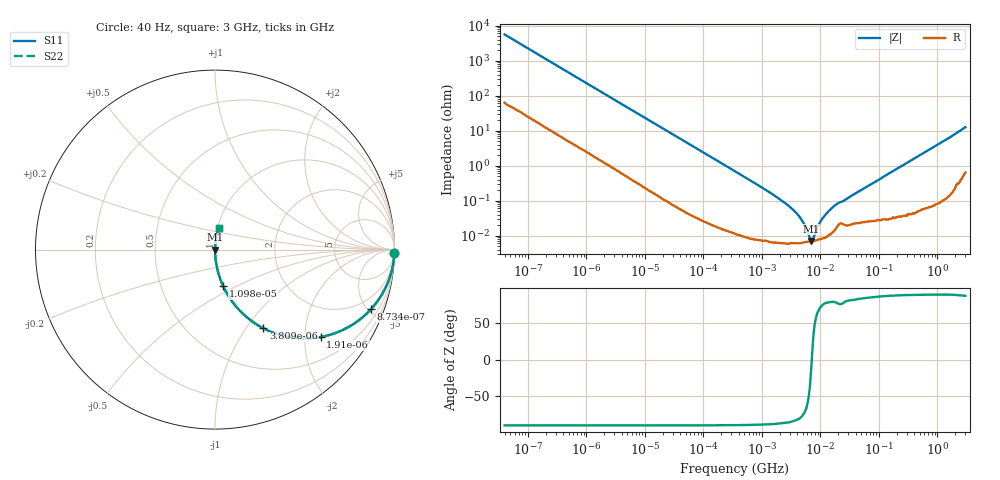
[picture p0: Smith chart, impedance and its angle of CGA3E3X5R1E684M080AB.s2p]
! S-parameter Generated by TDK Corporation
! Copyright(C) 2015 TDK Corporation.
! All Rights Reserved.
! TDK P/N: CGA3E3X5R1E684M080AB (Multilayer Ceramic Chip Capacitors)
! Property: C=680nF
! Size(LxWxT): 1.6x0.8x0.8mm, 0.063x0.031x0.031inches
! Model Type: s2p (Touchstone File Format Version 1.0)
! Frequency: DC=Yes Start=0.00004MHz Stop=3000MHz 396points Log-sweep
! Note: This model was converted from impedance.
! Model Generated on Jun. 23, 2015
! Hash(MD5):
! Port Assignments:
!  1 ---| |--- 2
! Applicable Conditions:
!  Temperature = 25 degC
!  DC Bias Voltage = 0 V
!  Small Signal Operation
! Terms and conditions regarding TDK Simulation Models
! (1)This simulation model is being provided solely for informational purposes. Please refer to the specifications of the products in terms of detailed characteristics of such products.
! (2)In no event shall TDK Corporation of any of its subsidiaries be liable for any loss or damage arising, directly or indirectly,
!  From any information contained in this simulation model, including, but not limited to loss or damages arising from any inaccuracies, omissions or errors in connection with such information.
! (3)Any and all copyrights on this simulation model are owned by TDK Corporation.
!  Duplication or redistribution of this simulation model without prior written permission from TDK Corporation is prohibited.
! (4)This simulation model is subject to any modification or change without any prior notice.
! (5)Neither TDK Corporation nor any of its subsidiaries shall make any warranty, express or implied,
!  Including but not limited to the correctness, implied warranties of merchantability and fitness for a particular purpose with respect to this simulation models.
! (6)The use of this simulation model shall be deemed to have consented to the terms and conditions hereof.
# MHz S MA R 50
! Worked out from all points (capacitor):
!   395 points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, 40 Hz to 3 GHz, reference 50 ohm
!   read as one part in series: C = 710 nF near 41.88 Hz
!   lowest |Z| = 6.98 mohm at 6.899 MHz (marker M1)
!   series resonance near 7.107 MHz, so ESL is about 710 pH
!   S11 on the Smith chart (normalised r, x): 40 Hz: open; 873.4 Hz: 1.06, -5.22; 1.91 kHz: 1.03, -2.40; 3.809 kHz: 1.01, -1.21; 10.98 kHz: 1.00, -0.42; 3 GHz: 1.01, +0.25
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4e-05  0.9996 -1.0  0.01783 88.3  0.01783 88.3  0.9996 -1.0
0.0002407527  0.9932 -6.1  0.1057 83.3  0.1057 83.3  0.9932 -6.1
0.000834128  0.9358 -20.0  0.3426 69.4  0.3426 69.4  0.9358 -20.0
0.000873414  0.9305 -20.9  0.3565 68.5  0.3565 68.5  0.9305 -20.9
0.001909884  0.7641 -39.6  0.6369 49.8  0.6369 49.8  0.7641 -39.6
0.003809071  0.515 -58.4  0.8519 31.0  0.8519 31.0  0.515 -58.4
0.006319477  0.3426 -69.4  0.936 20.0  0.936 20.0  0.3426 -69.4
0.01097819  0.2069 -77.5  0.9763 11.9  0.9763 11.9  0.2069 -77.5
0.01739424  0.133 -81.8  0.9898 7.6  0.9898 7.6  0.133 -81.8
0.3464102  0.006903 -88.7  0.9999 0.4  0.9999 0.4  0.006903 -88.7
2.877491  0.0007041 -85.2  0.9999 0.0  0.9999 0.0  0.0007041 -85.2
4.354128  0.0003502 -80.0  0.9999 0.0  0.9999 0.0  0.0003502 -80.0
5.480732  0.0001896 -69.9  0.9999 0.0  0.9999 0.0  0.0001896 -69.9
6.292177  0.0001072 -50.5  0.9999 0.0  0.9999 0.0  0.0001072 -50.5
6.898837  6.976e-05 -16.4  0.9999 0.0  0.9999 0.0  6.976e-05 -16.4
7.22376  6.992e-05 9.1  0.9999 -0.0  0.9999 -0.0  6.992e-05 9.1
7.920238  0.0001045 47.3  0.9999 -0.0  0.9999 -0.0  0.0001045 47.3
9.092863  0.0001877 65.7  0.9999 -0.0  0.9999 -0.0  0.0001877 65.7
10.93076  0.0003161 74.9  0.9999 -0.0  0.9999 -0.0  0.0003161 74.9
18.13479  0.0007563 78.3  0.9998 -0.0  0.9998 -0.0  0.0007563 78.3
150.6385  0.006067 86.8  0.9997 -0.3  0.9997 -0.3  0.006067 86.8
3000  0.1243 80.0  0.986 -7.1  0.986 -7.1  0.1243 80.0
